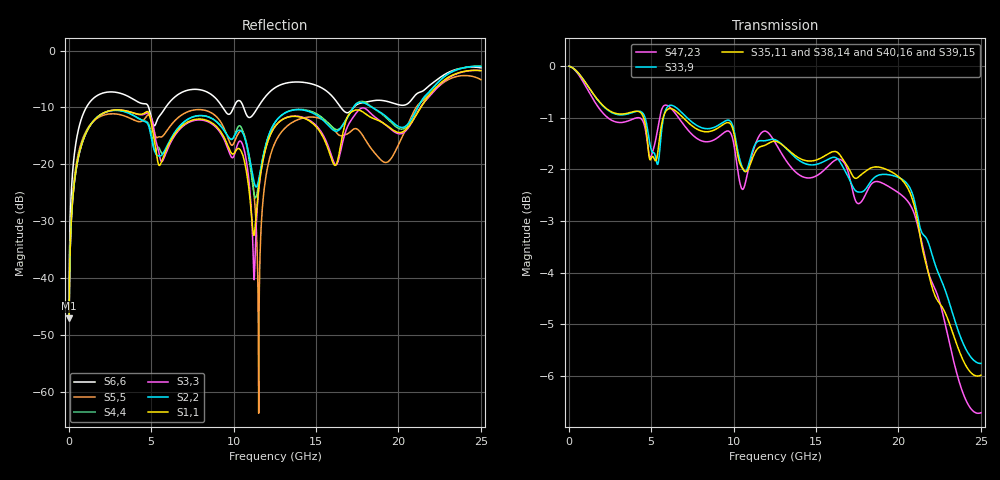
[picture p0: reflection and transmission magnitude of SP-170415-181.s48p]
! IMPORTANT NOTE: This model should not be used to evaluate
! electrical signals with a greater than 25 GHz. of frequency content.
! Please apply appropriate analysis techniques when reviewing the results of
! your simulations.
!  COPYRIGHT 2008, BY MOLEX INCORPORATED
!  ALL INTERNATIONAL RIGHTS RESERVED
!  THIS FILE CONTAINS MOLEX INCORPORATED CONFIDENTIAL INFORMATION
! >>>>>>>>>>>>>>>>  USER AGREEMENT  <<<<<<<<<<<<<<<<<<<
! The information on this media is the property of MOLEX Incorporated
! and  has been provided to you free of charge. Molex does not
! guarantee that the information is error-free, nor does MOLEX  make
! any representations, warranty or guarantee that the information is
! accurate, correct, reliable or up-to-date. MOLEX expressly
! disclaims all implied warranties regarding this information,
! including but not limited to any implied  warranties of
! merchantability or fitness for a particular purpose. MOLEX does
! not warrant that the media will work correctly in your multi- user
! or network environment.
! MOLEX will in no case be liable for your use, or the results of
! your use, of the software and other information contained on this
! media or  any accompanying written materials.  IT IS YOUR
! RESPONSIBILITY TO VERIFY THE RESULTS OF YOUR USE OF THIS
! INFORMATION IN YOUR OWN PARTICULAR ENGINEERING AND PRODUCT
! ENVIRONMENT, AND YOU ASSUME THE ENTIRE RISK OF DOING SO OR
! FAILING TO DO SO.  In no event will MOLEX be liable for any
! direct, indirect, incidental or consequential damages arising from
! your use of, or your inability to use, software, product simulations
! and other information contained on this media or any accompanying
! written materials.
! This model has not been validated with empirical data.
! This model was solved using HFSS.  TDR results can run 5-8 ohms low
! Touchstone file from project AM-170415-8018_rev7_30Oct
! Exported from HFSS 14.0.0
! Terminal data exported
! Port[1] = B1_T1
! Port[2] = C1_T1
! Port[3] = E1_T1
! Port[4] = F1_T1
! Port[5] = H1_T1
! Port[6] = J1_T1
! Port[7] = A2_T1
! Port[8] = B2_T1
! Port[9] = D2_T1
! Port[10] = E2_T1
! Port[11] = G2_T1
! Port[12] = H2_T1
! Port[13] = B3_T1
! Port[14] = C3_T1
! Port[15] = E3_T1
! Port[16] = F3_T1
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# GHZ S MA R 50.000000
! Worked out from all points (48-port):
!   1250 points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, 20 MHz to 25 GHz, reference 50 ohm
!   strongest paths, dB at 20 MHz, 6.26 GHz, 12.52 GHz, 18.76 GHz, 25 GHz:
!     S35,11: 0.0, -0.8, -1.5, -2.0, -6.0
!     S38,14: 0.0, -0.8, -1.5, -2.0, -6.2
!     S33,9: 0.0, -0.8, -1.4, -2.1, -5.8
!     S40,16: 0.0, -0.8, -1.5, -2.1, -6.1
!     S39,15: 0.0, -0.9, -1.6, -2.2, -5.4
!     S47,23: 0.0, -0.8, -1.5, -2.2, -6.7
!   lowest |S11| = -47.0 dB at 20 MHz (marker M1), VSWR 1.01, Z = 50 + j0.445 ohm
!   |S11| at or under -10 dB: start of sweep to 21.35 GHz
